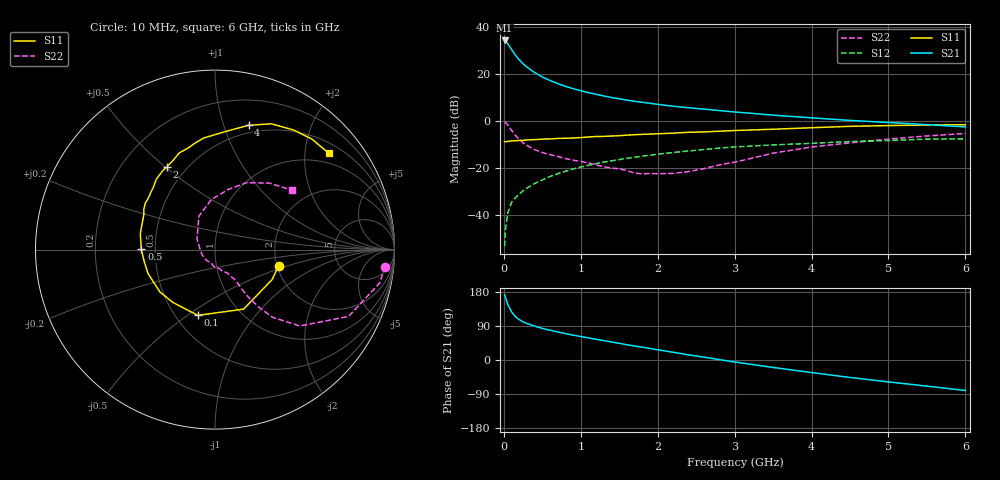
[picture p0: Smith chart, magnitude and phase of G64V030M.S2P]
! SIEMENS Small Signal Semiconductors
! BFG193
! Si NPN RF Bipolar Junction Transistor in SOT223
! VCE = 4 V  IC = 30 mA
! Common Emitter S-Parameters:  August  1996
# GHz  S  MA  R  50
!  f  S11  S21  S12  S22
! GHz  MAG  ANG  MAG  ANG  MAG  ANG  MAG  ANG
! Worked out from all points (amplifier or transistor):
!   36 points, 10 MHz to 6 GHz, reference 50 ohm
!   highest |S21| = 34.2 dB at 10 MHz (marker M1)
!   |S21| within 3 dB of that: start of sweep to 83.59 MHz
!   unconditionally stable (mu >= 1): 599.9 MHz to 2.388 GHz
!   at 250 MHz: K = 0.84, MSG = 27.0 dB, |S12| = -29.7 dB
!   at 1.4 GHz: K = 1.05, MAG = 12.1 dB, |S12| = -17.0 dB
!   at 6 GHz: K = 0.89, MSG = 2.5 dB, |S12| = -7.6 dB
!   S11 on the Smith chart (normalised r, x): 10 MHz: 2.04, -0.42; 100 MHz: 0.64, -0.55; 500 MHz: 0.42, +0.00; 2 GHz: 0.39, +0.51; 4 GHz: 0.43, +1.21; 6 GHz: 0.73, +2.53
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0.01  0.366 -14.1  51.01 172.3  0.0022 89.0  0.9541 -5.7
0.02  0.3594 -27.7  49.84 165.9  0.0047 85.7  0.9349 -11.6
0.05  0.3679 -64.3  43.74 147.0  0.0111 72.7  0.8321 -26.6
0.1  0.3786 -104.6  32.89 127.3  0.0186 64.8  0.6358 -42.0
0.15  0.3766 -128.7  24.85 114.3  0.0236 62.5  0.4939 -49.7
0.2  0.387 -142.4  19.87 106.6  0.0282 62.6  0.4077 -52.5
0.25  0.3878 -152.7  16.34 100.6  0.0328 63.2  0.3428 -54.4
0.3  0.3962 -160.4  13.88 96.2  0.0376 64.7  0.3034 -55.4
0.4  0.4008 -171.4  10.63 89.6  0.0468 65.3  0.2467 -55.9
0.5  0.4105 179.8  8.559 83.4  0.056 64.8  0.2133 -55.9
0.6  0.4154 173.9  7.213 78.6  0.0663 64.5  0.193 -56.9
0.8  0.4287 163.1  5.43 69.6  0.0857 61.9  0.1595 -60.8
1.1  0.4564 150.3  3.992 58.3  0.1144 57.5  0.1285 -70.7
1.6  0.4998 132.0  2.762 40.2  0.161 47.4  0.0882 -98.1
2  0.534 120.1  2.25 27.0  0.1966 38.8  0.0757 -140.1
2.2  0.5502 114.9  2.054 20.4  0.2142 34.3  0.0771 -157.3
2.8  0.6056 100.2  1.66 1.1  0.2649 20.6  0.1163 149.6
3.5  0.6664 83.6  1.327 -19.7  0.31 3.5  0.2071 115.6
4  0.7173 74.9  1.163 -33.1  0.3346 -6.2  0.2794 94.2
4.5  0.7678 65.9  1.026 -46.1  0.3653 -16.4  0.3423 77.8
5.5  0.8187 48.9  0.832 -68.9  0.4109 -39.6  0.4795 50.6
6  0.8305 40.4  0.748 -80.5  0.4175 -53.1  0.5419 37.6
